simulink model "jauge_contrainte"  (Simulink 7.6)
settings: Solver=ode15s  StartTime=0.0  StopTime=10.0  RelTol=1e-3
libraries: fl_lib x4, nesl_utility x4, elec_lib x3, simulink x1

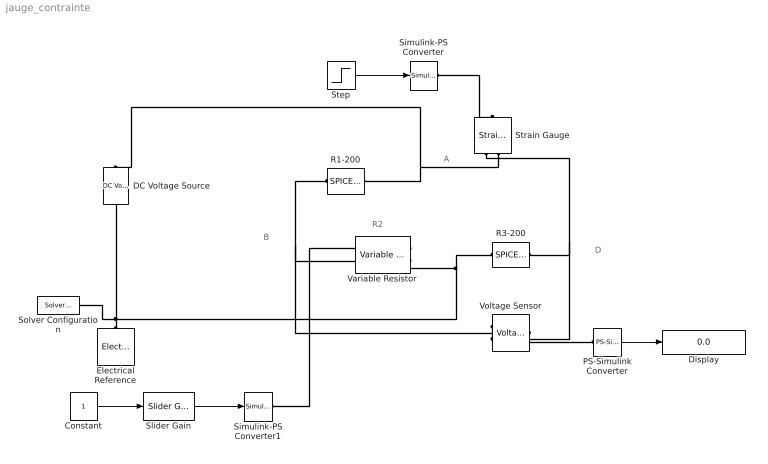
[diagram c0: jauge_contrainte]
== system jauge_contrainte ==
  note: A
  note: B
  note: D
  note: R2
  Constant : Constant
  DC Voltage Source : fl_lib/Electrical/Electrical Sources/DC Voltage Source  DialogController=NetworkEngine.DynNeDlgSource  SystemSampleTime=-1  v0=5 V  i_Log=off  v_Log=off  LocalVarNames=|i|v  LocalVarDescs=|i|v  LocalVarLogging=[0 0]
  Display : Display
  Electrical Reference : fl_lib/Electrical/Electrical Elements/Electrical Reference  DialogController=NetworkEngine.DynNeDlgSource  SystemSampleTime=-1  i_Log=off  LocalVarNames=|i  LocalVarDescs=|i  LocalVarLogging=0
  PS-Simulink Converter : nesl_utility/PS-Simulink Converter  DialogController=NetworkEngine.DynNeUtilDlgSource  SystemSampleTime=-1  PhysicalDomain=network_engine_domain  LeftPortType=input  RightPortType=output  SubClassName=ps_output  Unit=1  AffineConversion=off
  R1-200 : elec_lib/Additional Components/SPICE-Compatible Components/Passive Devices/SPICE Resistor  DialogController=NetworkEngine.DynNeDlgSource  SystemSampleTime=-1  SCALE=1  R_param=1  R=200 Ohm  RSH=0 Ohm  LENGTH=1e-06 m  WIDTH=1e-06 m  NARROW=0 m  T_param=1  TC1=0 1/K  TC2=0 1/K^2  TOFFSET=0 K  TFIXED=300.15 K  TMEAS=300.15 K  LocalVarLogging=[]
  R3-200 : elec_lib/Additional Components/SPICE-Compatible Components/Passive Devices/SPICE Resistor  DialogController=NetworkEngine.DynNeDlgSource  SystemSampleTime=-1  SCALE=1  R_param=1  R=200 Ohm  RSH=0 Ohm  LENGTH=1e-06 m  WIDTH=1e-06 m  NARROW=0 m  T_param=1  TC1=0 1/K  TC2=0 1/K^2  TOFFSET=0 K  TFIXED=300.15 K  TMEAS=300.15 K  LocalVarLogging=[]
  Simulink-PS Converter : nesl_utility/Simulink-PS Converter  DialogController=NetworkEngine.DynNeUtilDlgSource  SystemSampleTime=-1  PhysicalDomain=network_engine_domain  LeftPortType=input  RightPortType=output  SubClassName=ps_input  Unit=1  AffineConversion=off  InputFilterTimeConstant=.001  UdotUserProvided=0
  Simulink-PS Converter1 : nesl_utility/Simulink-PS Converter  DialogController=NetworkEngine.DynNeUtilDlgSource  SystemSampleTime=-1  PhysicalDomain=network_engine_domain  LeftPortType=input  RightPortType=output  SubClassName=ps_input  Unit=1  AffineConversion=off  InputFilterTimeConstant=.001  UdotUserProvided=0
  Slider Gain : simulink/Math Operations/Slider Gain  SystemSampleTime=-1  low=100  gain=133.4101  high=150
  Solver Configuration : nesl_utility/Solver Configuration  DialogController=NetworkEngine.DynNeUtilDlgSource  SystemSampleTime=-1  PhysicalDomain=network_engine_domain  LeftPortType=input  RightPortType=generic  SubClassName=solver  Accelerate=off  Profile=off  ResidualTolerance=1e-9  MaxNonlinIter=12  MaxModeIter=2  DoFixedCost=off  UseLocalSampling=off  DoDC=off  LinearAlgebra=Sparse  LocalSolverSampleTime=.001  LocalSolverChoice=NE_BACKWARD_EULER_ADVANCER  UseLocalSolver=off
  Step : Step  Time=2  SampleTime=0
  Strain Gauge : elec_lib/Sensors/Strain Gauge  DialogController=NetworkEngine.DynNeDlgSource  SystemSampleTime=-1  R=100 Ohm  K=2  current_Log=off  voltage_Log=off  power_Log=off  LocalVarNames=|current|voltage|power  LocalVarDescs=|Resistor current (A)|Voltage across resistor (V)|Power (W)  LocalVarLogging=[0 0 0]
  Variable Resistor : fl_lib/Electrical/Electrical Elements/Variable Resistor  DialogController=NetworkEngine.DynNeDlgSource  SystemSampleTime=-1  Rmin=0 Ohm  i_Log=off  v_Log=off  LocalVarNames=|i|v  LocalVarDescs=|i|v  LocalVarLogging=[0 0]
  Voltage Sensor : fl_lib/Electrical/Electrical Sensors/Voltage Sensor  DialogController=NetworkEngine.DynNeDlgSource  SystemSampleTime=-1  i1_Log=off  v1_Log=off  LocalVarNames=|i1|v1  LocalVarDescs=|i1|v1  LocalVarLogging=[0 0]
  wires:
  PS-Simulink Converter/1 -> Display/1
  Step/1 -> Simulink-PS Converter/1
  Slider Gain/1 -> Simulink-PS Converter1/1
  Constant/1 -> Slider Gain/1
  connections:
  Strain Gauge/RConn2 -- R1-200/LConn1 -- DC Voltage Source/LConn1
  R1-200/RConn1 -- Voltage Sensor/LConn1 -- Variable Resistor/LConn2
  Strain Gauge/RConn1 -- Voltage Sensor/RConn2 -- R3-200/LConn1
  Voltage Sensor/RConn1 -- PS-Simulink Converter/LConn1
  Simulink-PS Converter/RConn1 -- Strain Gauge/LConn1
  Electrical Reference/LConn1 -- Variable Resistor/RConn1 -- R3-200/RConn1 -- DC Voltage Source/RConn1 -- Solver Configuration/RConn1
  Simulink-PS Converter1/RConn1 -- Variable Resistor/LConn1
